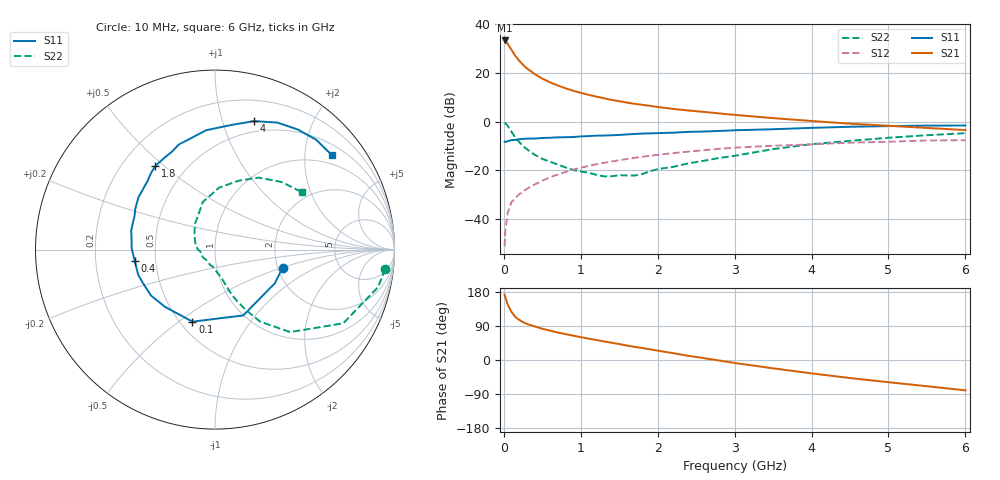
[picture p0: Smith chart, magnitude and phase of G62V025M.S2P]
! SIEMENS Small Signal Semiconductors
! BFG193
! Si NPN RF Bipolar Junction Transistor in SOT223
! VCE = 2 V  IC = 25 mA
! Common Emitter S-Parameters:  August  1996
# GHz  S  MA  R  50
!  f  S11  S21  S12  S22
! GHz  MAG  ANG  MAG  ANG  MAG  ANG  MAG  ANG
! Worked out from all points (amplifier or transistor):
!   36 points, 10 MHz to 6 GHz, reference 50 ohm
!   highest |S21| = 33.3 dB at 10 MHz (marker M1)
!   |S21| within 3 dB of that: start of sweep to 82.41 MHz
!   unconditionally stable (mu >= 1): 605.1 MHz to 2.638 GHz
!   at 250 MHz: K = 0.81, MSG = 26.0 dB, |S12| = -28.6 dB
!   at 1.4 GHz: K = 1.05, MAG = 11.2 dB, |S12| = -16.3 dB
!   at 6 GHz: K = 0.92, MSG = 2.1 dB, |S12| = -7.6 dB
!   S11 on the Smith chart (normalised r, x): 10 MHz: 2.12, -0.51; 100 MHz: 0.58, -0.56; 400 MHz: 0.38, -0.06; 1.8 GHz: 0.34, +0.47; 4 GHz: 0.39, +1.27; 6 GHz: 0.74, +2.63
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0.01  0.3898 -15.2  46.44 172.4  0.0028 89.4  0.9552 -6.5
0.02  0.3824 -29.5  45.37 165.6  0.0059 80.3  0.9318 -13.0
0.05  0.3991 -66.8  39.72 146.4  0.0135 69.6  0.824 -29.9
0.1  0.4207 -107.4  29.67 126.7  0.0224 62.2  0.6211 -47.7
0.15  0.4236 -131.2  22.34 113.5  0.0274 58.3  0.4737 -57.9
0.2  0.4389 -144.3  17.85 105.9  0.0325 59.3  0.3829 -62.6
0.25  0.4427 -155.1  14.65 99.8  0.0371 59.4  0.3144 -66.6
0.3  0.4502 -161.8  12.44 95.3  0.042 60.9  0.2733 -69.3
0.4  0.452 -172.2  9.509 88.7  0.0516 61.7  0.2107 -73.0
0.5  0.4645 179.0  7.655 82.4  0.0616 61.4  0.1732 -75.7
0.6  0.4682 173.3  6.438 77.5  0.0726 61.3  0.1512 -78.8
0.7  0.4786 167.3  5.551 72.6  0.0825 60.6  0.1328 -83.5
0.9  0.4857 157.5  4.329 64.2  0.1039 57.7  0.1027 -92.4
1.1  0.5069 149.2  3.562 56.6  0.1237 54.7  0.0899 -108.0
1.4  0.5276 138.1  2.806 45.6  0.1525 48.8  0.0761 -136.6
1.8  0.5718 125.6  2.222 31.6  0.1912 40.6  0.0846 -174.1
2.2  0.5957 113.8  1.833 18.0  0.2271 31.1  0.1185 158.9
3.5  0.7014 82.3  1.185 -22.0  0.3217 0.0  0.2744 104.2
4  0.748 73.1  1.035 -35.3  0.3431 -9.7  0.3454 86.3
4.5  0.7883 63.9  0.911 -47.6  0.3716 -19.7  0.405 71.3
5.5  0.832 47.4  0.746 -69.2  0.4129 -42.7  0.5288 45.5
6  0.8372 39.1  0.674 -80.1  0.4166 -55.8  0.582 33.2
